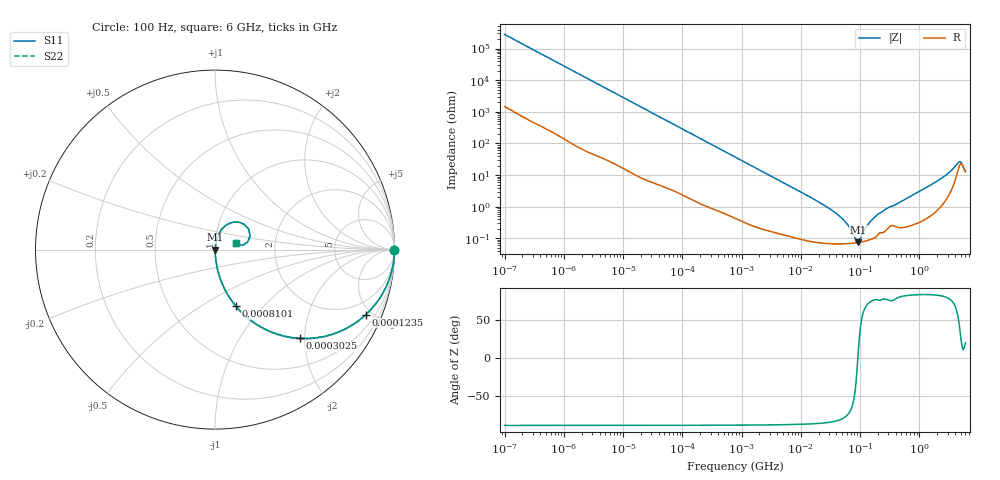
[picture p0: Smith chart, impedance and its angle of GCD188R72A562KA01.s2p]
!Murata Part Number: GCD188R72A562KA01
!These Parameters are Measured in Series Mode Connection
!Data Generated on Mar 13, 2026
!  o--ll--o
!Port1  Port2
!  o------o
!Operation Temp=25[degC], DC Bias Voltage=0[V]
!Freq. Start=100[Hz] Stop=6[GHz] 401[Steps]
# Hz S RI R 50
!Freq.(Hz) S11(Real) S11(Imag) S21(Real) S21(Imag) S12(Real) S12(Imag) S22(Real) S22(Imag)
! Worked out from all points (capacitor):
!   401 points, 100 Hz to 6 GHz, reference 50 ohm
!   read as one part in series: C = 5.7 nF near 109 Hz
!   lowest |Z| = 74.3 mohm at 93.27 MHz (marker M1)
!   series resonance near 91.8 MHz, so ESL is about 530 pH
!   S11 on the Smith chart (normalised r, x): 100 Hz: open; 123.5 kHz: 1.04, -4.63; 302.5 kHz: 1.02, -1.90; 810.1 kHz: 1.01, -0.71; 6 GHz: 1.25, +0.09
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100  1 -0.000359  2e-06 0.000359  2e-06 0.000359  1 -0.000359
2008  0.9999 -0.00713  8.45e-05 0.00713  8.45e-05 0.00713  0.9999 -0.00713
12592  0.9978 -0.0443  0.00222 0.0443  0.00222 0.0443  0.9978 -0.0443
40335  0.9794 -0.1388  0.0206 0.1388  0.0206 0.1388  0.9794 -0.1388
123542  0.8407 -0.3618  0.1593 0.3618  0.1593 0.3618  0.8407 -0.3618
302498  0.4745 -0.4946  0.5255 0.4946  0.5255 0.4946  0.4745 -0.4946
774597  0.1251 -0.3251  0.8749 0.3251  0.8749 0.3251  0.1251 -0.3251
810067  0.1158 -0.3143  0.8842 0.3143  0.8842 0.3143  0.1158 -0.3143
2837864  0.0121 -0.1012  0.9879 0.1012  0.9879 0.1012  0.0121 -0.1012
1.555665e7  0.00112 -0.0184  0.9989 0.0184  0.9989 0.0184  0.00112 -0.0184
4.764863e7  0.000687 -0.00454  0.9993 0.00454  0.9993 0.00454  0.000687 -0.00454
6.518806e7  0.000688 -0.00225  0.9993 0.00225  0.9993 0.00225  0.000688 -0.00225
8.527865e7  0.000718 -0.000474  0.9993 0.000474  0.9993 0.000474  0.000718 -0.000474
9.326766e7  0.000735 0.000104  0.9993 -0.000104  0.9993 -0.000104  0.000735 0.000104
1.275994e8  0.000835 0.00216  0.9992 -0.00216  0.9992 -0.00216  0.000835 0.00216
1.526266e8  0.000937 0.00343  0.9991 -0.00343  0.9991 -0.00343  0.000937 0.00343
1.996653e8  0.0013 0.00558  0.9987 -0.00558  0.9987 -0.00558  0.0013 0.00558
3.124326e8  0.00236 0.00939  0.9976 -0.00939  0.9976 -0.00939  0.00236 0.00939
2.679998e9  0.0221 0.0888  0.9779 -0.0888  0.9779 -0.0888  0.0221 0.0888
4.586474e9  0.1611 0.1421  0.8389 -0.1421  0.8389 -0.1421  0.1611 0.1421
5.016141e9  0.196 0.0776  0.804 -0.0776  0.804 -0.0776  0.196 0.0776
6e9  0.1146 0.0366  0.8854 -0.0366  0.8854 -0.0366  0.1146 0.0366
